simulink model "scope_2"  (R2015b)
settings: Solver=ode45  StartTime=0.0  StopTime=10.0  RelTol=1e-3
undefined symbols (not defined in the file or in its folder): fir1

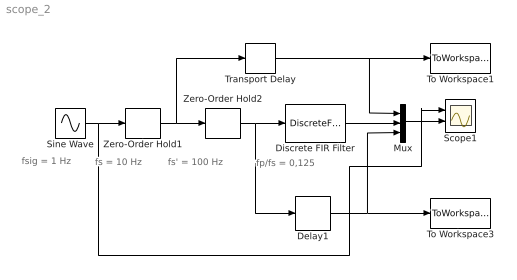
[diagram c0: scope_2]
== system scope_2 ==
  note: fsig = 1 Hz
  note: fp/fs = 0,125
  note: fs' = 100 Hz
  note: fs = 10 Hz
  Delay1 : Delay  DelayLength=64
  Discrete FIR Filter : DiscreteFir  Coefficients=fir1(128,0.025)
  Mux : Mux  Inputs=3
  Scope1 : Scope  NumInputPorts=2
  Sine Wave : Sin  Frequency=2*pi*1  SampleTime=0
  To Workspace1 : ToWorkspace  VariableName=y2  SaveFormat=Timeseries  SampleTime=-1
  To Workspace3 : ToWorkspace  VariableName=y1  SaveFormat=Timeseries  SampleTime=-1
  Transport Delay : TransportDelay  DelayTime=0.64
  Zero-Order Hold1 : ZeroOrderHold  SampleTime=1/10
  Zero-Order Hold2 : ZeroOrderHold  SampleTime=1/100
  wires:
  Mux/1 -> Scope1/2
  Sine Wave/1 -> Scope1/1, Zero-Order Hold1/1
  Zero-Order Hold2/1 -> Delay1/1, Discrete FIR Filter/1
  Delay1/1 -> To Workspace3/1, Mux/3
  Discrete FIR Filter/1 -> Mux/2
  Zero-Order Hold1/1 -> Transport Delay/1, Zero-Order Hold2/1
  Transport Delay/1 -> Mux/1, To Workspace1/1
